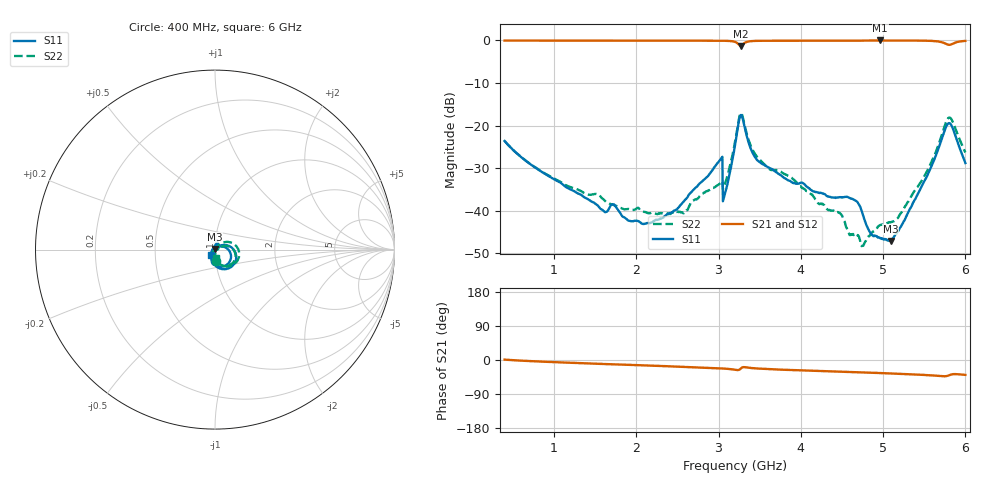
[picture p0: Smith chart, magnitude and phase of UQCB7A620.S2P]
!  Part Number  UQCB7A620	Mounting Orientation: Vertical
!  Description: RF capacitors
!  Application: Coupling, Bypass, Tuning, DC Block
!  Filters, Matching
# GHZ S DB R 50
! Freq  |S11|  S11 Ph  |S21|  S21 Ph  |S12|  S12 Ph  |S22|  S22 Ph
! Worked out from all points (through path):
!   801 points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, 400 MHz to 6 GHz, reference 50 ohm
!   highest |S21| = 0.00 dB at 4.964 GHz (marker M1); lowest = -1.3 dB at 3.27 GHz (marker M2)
!   group delay of S21, straight-line fit = 20.2 ps
!   lowest |S11| = -47.1 dB at 5.09 GHz (marker M3), VSWR 1.01, Z = 49.9 + j0.425 ohm
!   |S11| at or under -10 dB: start of sweep to end of sweep
!   |S22| runs from -48.3 to -17.1 dB; largest |S21 - S12| = 0.0025
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0.4  -23.60 -88.7  -0.03 1.0  -0.04 1.0  -23.59 -86.9
1.338  -36.37 -110.3  -0.03 -8.4  -0.04 -8.4  -35.46 -80.8
1.73  -38.50 -131.6  -0.04 -11.5  -0.05 -11.5  -38.69 -71.8
1.926  -42.39 -154.4  -0.03 -12.9  -0.04 -12.9  -39.62 -59.0
2.269  -42.06 156.9  -0.03 -15.6  -0.04 -15.6  -40.62 -37.2
2.591  -37.47 117.4  -0.03 -18.1  -0.04 -18.1  -40.20 -6.4
3.018  -28.07 70.4  -0.07 -22.0  -0.08 -22.0  -33.58 23.8
3.081  -35.81 41.8  -0.08 -22.9  -0.09 -22.8  -33.48 49.6
3.2  -24.60 26.2  -0.33 -25.7  -0.34 -25.6  -23.89 39.3
3.27  -17.50 -35.6  -1.32 -22.6  -1.32 -22.6  -17.07 -17.5
3.473  -28.16 -113.5  -0.09 -22.5  -0.10 -22.4  -27.43 -91.6
4.138  -35.27 -156.1  -0.08 -28.2  -0.09 -28.1  -36.16 -131.7
4.474  -36.81 -166.5  -0.06 -30.7  -0.06 -30.6  -40.47 -122.1
4.628  -37.20 171.8  -0.05 -31.8  -0.06 -31.7  -45.61 -101.6
4.747  -40.50 140.8  -0.04 -32.6  -0.04 -32.5  -48.20 -78.1
4.852  -45.33 140.0  -0.01 -33.5  -0.01 -33.4  -45.35 -47.9
4.964  -46.45 131.1  0.00 -34.5  -0.01 -34.4  -43.35 -36.3
5.069  -46.97 109.6  -0.01 -35.4  -0.01 -35.3  -42.73 -26.5
5.09  -47.10 105.5  -0.01 -35.6  -0.01 -35.5  -42.72 -22.3
5.517  -32.48 40.6  -0.06 -39.6  -0.06 -39.5  -31.28 23.7
5.783  -19.65 -35.0  -0.95 -41.7  -0.95 -41.6  -18.45 -16.7
6  -28.78 -127.5  -0.11 -39.2  -0.10 -39.1  -26.29 -83.6
